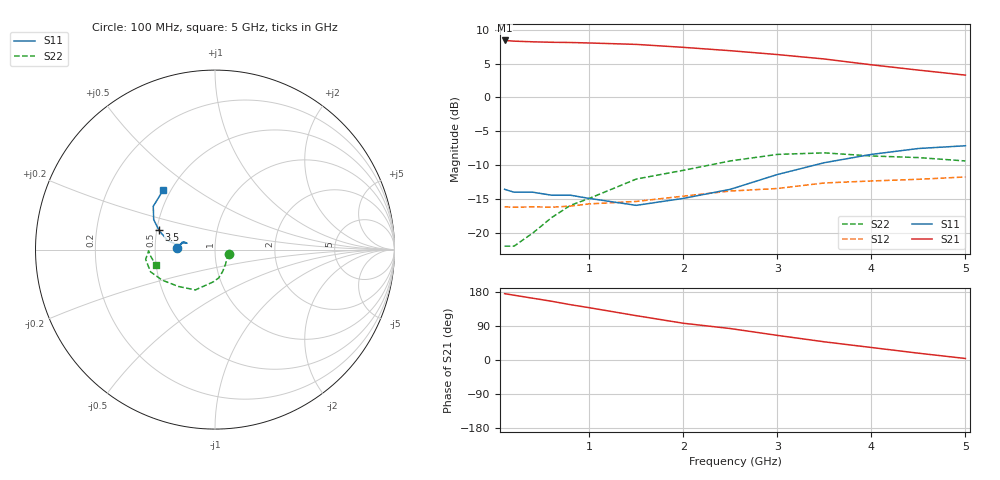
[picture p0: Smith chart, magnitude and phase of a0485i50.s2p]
!  MSA-0485 S AND NOISE PARAMETERS
!  Id=50mA  LAST UPDATED 07-22-92
# ghz s ma r 50
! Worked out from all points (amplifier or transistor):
!   14 points, 100 MHz to 5 GHz, reference 50 ohm
!   highest |S21| = 8.4 dB at 100 MHz (marker M1)
!   |S21| within 3 dB of that: start of sweep to 3.656 GHz
!   unconditionally stable (mu >= 1): start of sweep to end of sweep
!   at 400 MHz: K = 1.37, MAG = 8.5 dB, |S12| = -16.1 dB
!   at 2 GHz: K = 1.22, MAG = 8.2 dB, |S12| = -14.6 dB
!   at 5 GHz: K = 1.01, MAG = 6.9 dB, |S12| = -11.7 dB
!   lowest NFmin = 6.70 dB at 100 MHz
!   S11 on the Smith chart (normalised r, x): 100 MHz: 0.65, +0.02; 3.5 GHz: 0.51, +0.12; 5 GHz: 0.46, +0.38
0.1  0.21 177.0  2.63 175.0  0.156 2.0  0.08 -16.0
0.2  0.2 176.0  2.6 171.0  0.155 2.0  0.08 -30.0
0.4  0.2 172.0  2.57 163.0  0.156 3.0  0.1 -54.0
0.6  0.19 171.0  2.55 155.0  0.155 5.0  0.13 -71.0
0.8  0.19 168.0  2.54 146.0  0.158 6.0  0.16 -83.0
1  0.18 166.0  2.52 138.0  0.164 9.0  0.18 -93.0
1.5  0.16 167.0  2.46 117.0  0.171 11.0  0.25 -116.0
2  0.18 168.0  2.34 97.0  0.187 12.0  0.29 -135.0
2.5  0.21 173.0  2.21 83.0  0.204 16.0  0.34 -150.0
3  0.27 169.0  2.07 65.0  0.213 13.0  0.38 -161.0
3.5  0.33 161.0  1.92 48.0  0.234 9.0  0.39 -172.0
4  0.38 154.0  1.74 33.0  0.242 6.0  0.37 -179.0
4.5  0.42 145.0  1.59 18.0  0.249 3.0  0.36 -174.0
5  0.44 131.0  1.46 4.0  0.259 -3.0  0.34 -165.0
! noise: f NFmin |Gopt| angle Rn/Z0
0.1  6.7  0.12  -179  0.65
0.5  6.7  0.13  -175  0.65
1  7  0.14  -170  0.65
2  7.7  0.2  -154  0.65
